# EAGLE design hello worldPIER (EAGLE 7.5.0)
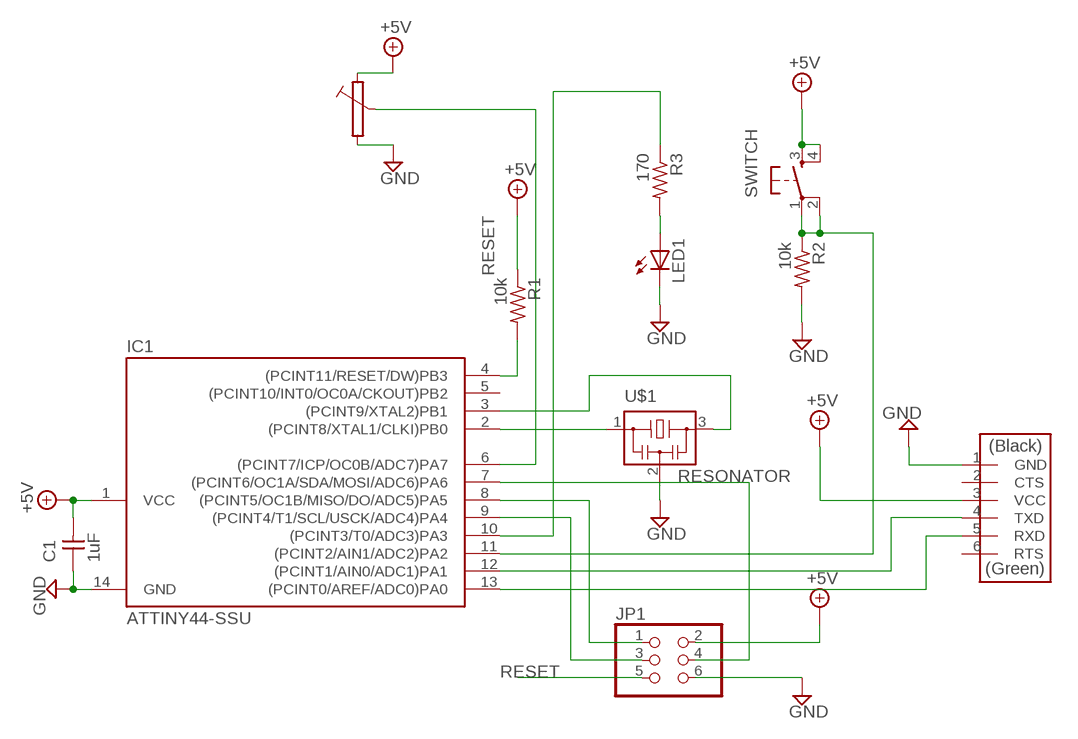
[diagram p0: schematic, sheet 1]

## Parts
C1  1uF  CAP-UNPOLARIZEDFAB  [C1206FAB]
IC1  ATTINY44-SSU  [SOIC14]
JP1  PINHD-2X3-SMD  [2X03SMD]
LED1  LEDP-LCC-2  [P-LCC-2]
R1  10k  RES-US1206FAB  [R1206FAB]
R2  10k  RES-US1206FAB  [R1206FAB]
R3  170  RES-US1206FAB  [R1206FAB]
SWITCH  6MM_SWITCH6MM_SWITCH  [6MM_SWITCH]
U$1  RESONATOR  [EFOBM]
U$2  FTDI-SMD-HEADER  [1X06SMD]

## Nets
+5V: C1.2 IC1.1(VCC) JP1.2 R1.1 SWITCH.3(S) SWITCH.4(S1) U$2.3(VCC)
GND: C1.1 IC1.14(GND) JP1.6 LED1.C R2.2 U$1.2 U$2.1(GND)
N$1: IC1.2((PCINT8/XTAL1/CLKI)PB0) U$1.1
N$2: IC1.3((PCINT9/XTAL2)PB1) U$1.3
N$3: IC1.12((PCINT1/AIN0/ADC1)PA1) U$2.4(TXD)
N$4: IC1.8((PCINT5/OC1B/MISO/DO/ADC5)PA5) JP1.1
N$5: IC1.7((PCINT6/OC1A/SDA/MOSI/ADC6)PA6) JP1.4
N$6: IC1.9((PCINT4/T1/SCL/USCK/ADC4)PA4) JP1.3
N$7: IC1.13((PCINT0/AREF/ADC0)PA0) U$2.5(RXD)
N$8: IC1.11((PCINT2/AIN1/ADC2)PA2) R2.1 SWITCH.1(P) SWITCH.2(P1)
N$9: IC1.6((PCINT7/ICP/OC0B/ADC7)PA7)
N$10: LED1.A R3.2
N$11: IC1.10((PCINT3/T0/ADC3)PA3) R3.1
RESET: IC1.4((PCINT11/RESET/DW)PB3) JP1.5 R1.2
Unconnected: IC1.5((PCINT10/INT0/OC0A/CKOUT)PB2) U$2.2(CTS) U$2.6(RTS)

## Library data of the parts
C1 = fab:CAP-UNPOLARIZED
IC1 = fab:ATTINY44
JP1 = fab:PINHD-2X3-SMD: PIN HEADER
LED1 = adafruit:LED: LED
R1-R3 = fab:RES-US: Resistor (US Symbol)
SWITCH = fab:6MM_SWITCH: OMRON SWITCH
U$1 = fab:RESONATOR
U$2 = fab:FTDI-SMD-HEADER

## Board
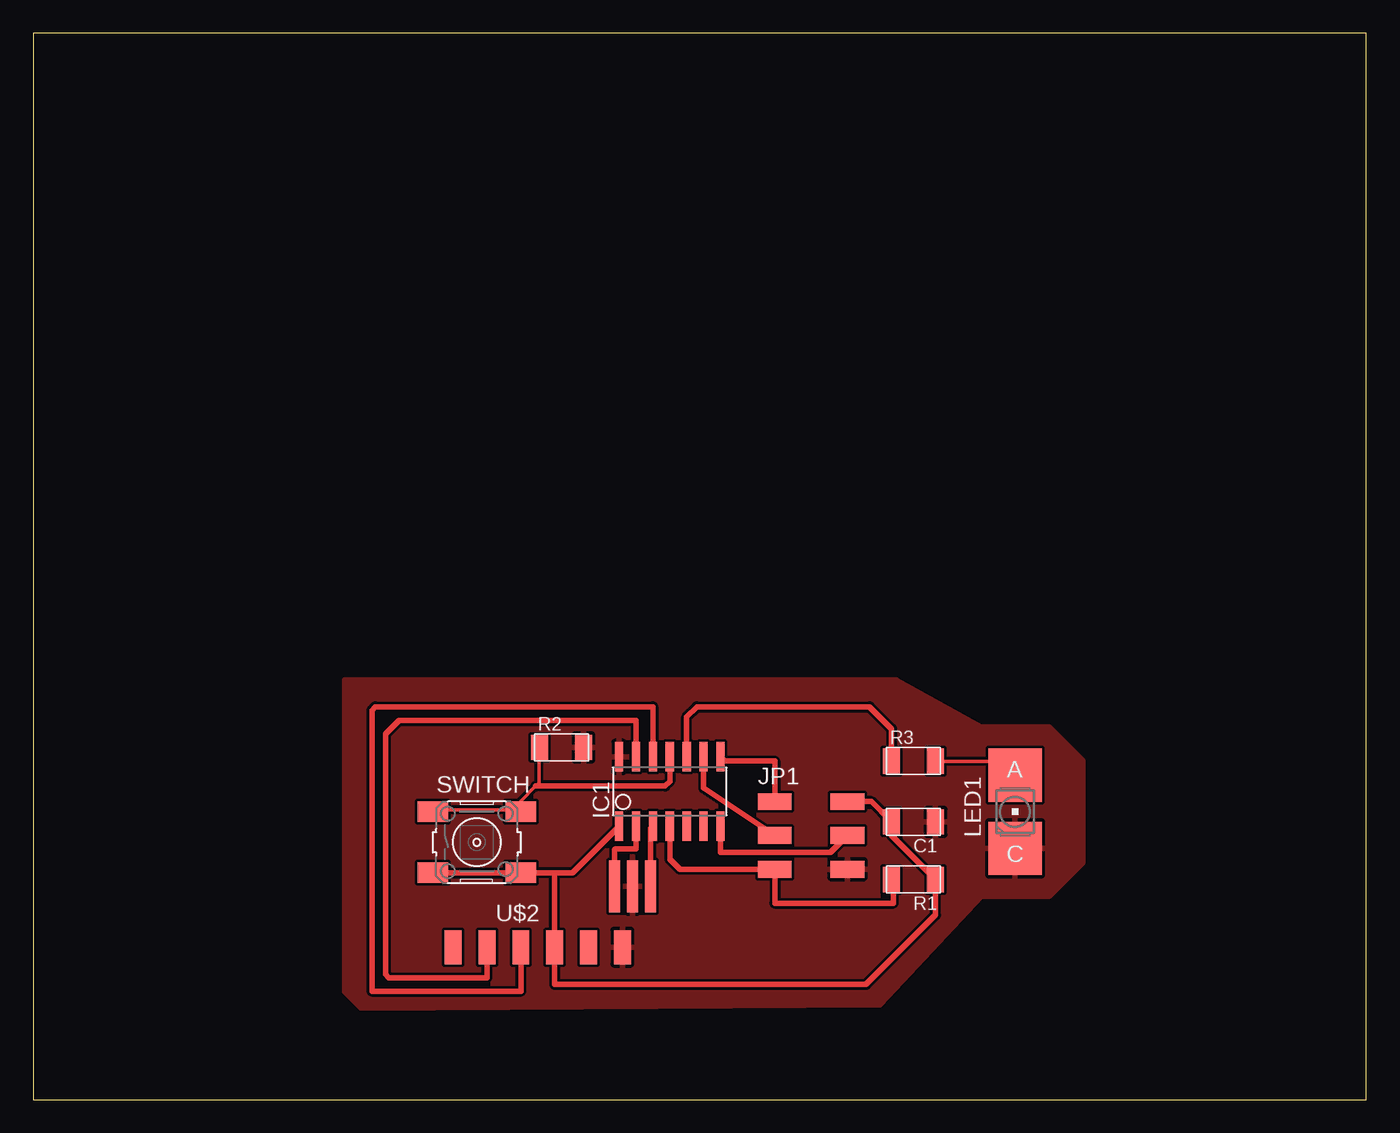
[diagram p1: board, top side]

Size 100 x 80 mm. Coordinates in mm from the lower left corner, seen from the top.
Outline: 0,0 100,0 100,80 0,80 0,0
Copper layers (1*16): Top 0.035mm / dielectric 1.5mm / Bottom 0.035mm
Design rules "default": minimum track width 10mil, minimum drill 24mil, track to track 8mil, track to pad 8mil, pad to pad 8mil, via to via 8mil, smd to smd 8mil, copper to edge 40mil, drill to drill 8mil, minimum pad ring 10mil, minimum via ring 8mil, stop-mask expansion 4mil, vias tented up to drill 0mil, thermal gap 10mil

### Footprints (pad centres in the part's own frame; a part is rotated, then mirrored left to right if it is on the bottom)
C1206FAB = smd 1.27 x 1.905: 1 -1.651,0; 2 1.651,0
SOIC14 = smd 0.61 x 2.21: 1 -3.81,-2.603; 2 -2.54,-2.603; 3 -1.27,-2.603; 4 0,-2.603; 5 1.27,-2.603; 6 2.54,-2.603; 7 3.81,-2.603; 8 3.81,2.603; 9 2.54,2.603; 10 1.27,2.603; 11 0,2.603; 12 -1.27,2.603; 13 -2.54,2.603; 14 -3.81,2.603
2X03SMD = smd 2.54 x 1.27: 1 -2.54,2.54; 2 2.92,2.54; 3 -2.54,0; 4 2.92,0; 5 -2.54,-2.54; 6 2.92,-2.54
P-LCC-2 = smd 4 x 4: A 0,2.75; C 0,-2.75
R1206FAB = smd 1.27 x 1.905: 1 -1.651,0; 2 1.651,0
6MM_SWITCH = smd 2.286 x 1.524: 1 -3.302,2.286; 2 3.302,2.286; 3 -3.302,-2.286; 4 3.302,-2.286
EFOBM = smd 0.8 x 3.9: 1 -1.35,0; 2 0,0; 3 1.35,0
1X06SMD = smd 2.54 x 1.27: 1 0,6.35; 2 0,3.81; 3 0,1.27; 4 0,-1.27; 5 0,-3.81; 6 0,-6.35

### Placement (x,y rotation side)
C1  66.04,20.83 180 top
IC1  47.75,23.11 0 top
JP1  58.17,19.81 0 top
LED1  73.66,21.59 0 top
R1  66.04,16.51 180 top
R2  39.62,26.42 0 top
R3  66.04,25.4 0 top
SWITCH  33.27,19.3 0 top
U$1  44.96,16 0 top
U$2  37.85,11.43 270 top

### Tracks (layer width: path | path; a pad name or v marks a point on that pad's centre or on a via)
+5V
  Top 0.406: SWITCH.3 SWITCH.4 39.12,17.02 | IC1.1 40.45,17.02 39.12,17.02 | JP1.2 62.87,22.35 C1.2 64.39,19.81 R1.1 67.69,13.84 62.48,8.64 39.12,8.64 U$2.3 39.12,17.02
GND
  pour Top: 23.37,31.5 64.77,31.5 71.12,27.94 76.2,27.94 78.74,25.4 78.74,17.78 76.2,15.24 71.12,15.24 63.5,7.11 24.64,6.86 23.37,8.13
N$1
  Top 0.406: IC1.2 45.21,18.8 43.69,18.8 43.61,18.72 U$1.1
N$2
  Top 0.406: IC1.3 46.31,20.34 U$1.3
N$3
  Top 0.406: IC1.12 46.48,29.46 25.65,29.46 25.4,29.21 25.4,8.13 36.58,8.13 U$2.4
N$4
  Top 0.406: IC1.8 51.88,25.4 55.63,25.4 JP1.1
N$5
  Top 0.406: JP1.4 59.82,18.54 51.56,18.54 IC1.7
N$6
  Top 0.406: IC1.9 50.29,23.37 JP1.3
N$7
  Top 0.406: IC1.13 45.21,28.45 27.43,28.45 26.42,27.43 26.42,9.4 26.67,9.14 34.04,9.14 U$2.5
N$8
  Top 0.254: 36.58,21.72 36.58,22.4 37.69,23.52 37.95,23.77 37.95,26.29 R2.1 | 36.58,21.72 30.18,21.72 SWITCH.1 | 36.58,21.72 SWITCH.2
  Top 0.406: IC1.11 47.75,23.88 47.4,23.52 37.69,23.52
N$10
  Top 0.254: R3.2 67.89,25.38 72.69,25.38 73.61,24.46 LED1.A
N$11
  Top 0.406: IC1.10 49.02,28.7 49.78,29.46 62.74,29.46 64.39,27.81 R3.1
RESET
  Top 0.406: R1.2 64.52,16.51 64.52,14.73 55.63,14.73 JP1.5 48.51,17.27 47.75,18.03 IC1.4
